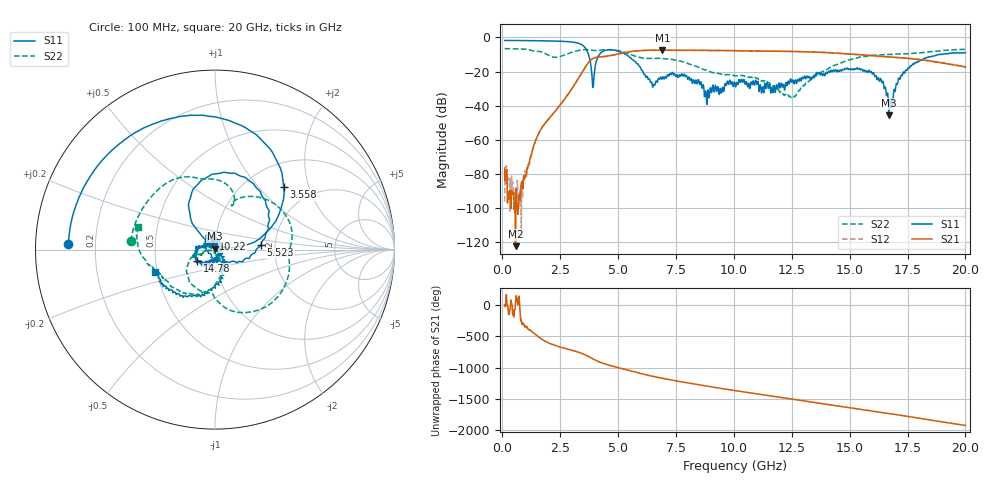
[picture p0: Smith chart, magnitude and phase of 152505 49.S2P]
!  2-Port S-parameters saved by WinCal
! VAR MeasName=S-Parameters (CALIBRATED_DATA) read from VNA (N5230C)
! VAR MeasDate=4/10/2015 9:33:28 AM
! VAR NAME=152505 49
! VAR FILENAME=152505 49.S2P
! VAR DATE=4/10/2015 9:33:28 AM
! VAR PHYS_PORTS=1,2
# Hz S DB R 50
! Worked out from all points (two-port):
!   801 points, 100 MHz to 20 GHz, reference 50 ohm
!   highest |S21| = -7.42 dB at 6.916 GHz (marker M1); lowest = -122.4 dB at 572.6 MHz (marker M2)
!   |S21| within 3 dB of the highest: 4.749 GHz to 15.76 GHz (11.01 GHz wide, 107 % of centre)
!   lowest |S11| = -45.7 dB at 16.69 GHz (marker M3), VSWR 1.01, Z = 50 + j0.52 ohm
!   |S11| at or under -10 dB: 3.722 GHz to 4.194 GHz (471.9 MHz wide, 11.9 % of centre); 5.35 GHz to 18.84 GHz (13.49 GHz wide, 112 % of centre); 18.89241 GHz to 18.91252 GHz (20.12 MHz wide, 0.106 % of centre)
!   |S22| runs from -35.6 to -6.5 dB; largest |S21 - S12| = 0.0065
!   S11 on the Smith chart (normalised r, x): 100 MHz: 0.10, +0.02; 3.558 GHz: 1.45, +1.39; 5.523 GHz: 1.68, +0.09; 10.22 GHz: 0.97, +0.11; 14.78 GHz: 0.81, -0.10; 20 GHz: 0.49, -0.14
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1e8  -1.75 177.7  -76.58 4.5  -96.25 114.4  -6.55 174.3
5.72625e8  -1.78 166.4  -122.41 25.7  -88.99 124.5  -6.69 147.4
9.955e8  -1.83 156.1  -80.54 30.1  -77.94 16.2  -6.84 121.9
1.64225e9  -1.94 139.3  -54.45 -172.7  -54.60 -172.8  -8.29 85.8
3.43325e9  -4.25 56.9  -20.67 -53.4  -20.70 -53.4  -7.26 29.5
3.557625e9  -5.71 42.4  -17.90 -72.4  -17.92 -72.4  -7.09 21.0
3.93075e9  -28.74 107.6  -12.25 -145.1  -12.27 -145.2  -7.63 -0.0
4.3785e9  -7.95 98.0  -11.19 145.3  -11.25 144.9  -7.25 -19.7
5.52275e9  -11.80 5.5  -8.31 27.5  -8.33 27.5  -9.90 -81.8
6.741625e9  -23.90 169.7  -7.45 -77.7  -7.44 -77.9  -12.22 -107.6
6.91575e9  -23.72 149.2  -7.42 -90.6  -7.46 -90.6  -12.35 -113.0
8.30875e9  -27.10 75.7  -7.56 176.3  -7.57 176.5  -16.55 -158.5
8.831125e9  -39.33 77.0  -7.57 144.0  -7.61 144.1  -19.24 -164.1
1.005e10  -26.89 127.1  -7.73 73.1  -7.76 73.1  -22.42 -160.2
1.022412e10  -24.61 100.9  -7.80 63.3  -7.78 63.7  -22.19 -160.2
1.248775e10  -25.90 -64.0  -8.19 -61.6  -8.24 -61.3  -35.58 -108.3
1.338325e10  -23.19 -106.8  -8.53 -110.9  -8.48 -110.8  -24.02 -65.1
1.477625e10  -18.58 -147.8  -9.50 171.5  -9.49 171.1  -14.11 -90.2
1.594538e10  -20.12 174.8  -10.63 107.3  -10.62 107.3  -10.57 -123.7
1.669162e10  -45.67 92.6  -11.37 67.2  -11.41 67.0  -9.93 -141.1
1.7811e10  -14.87 -81.0  -12.66 3.6  -12.62 3.4  -9.27 -159.3
2e10  -8.98 -159.9  -17.28 -123.2  -17.23 -123.0  -6.99 163.6
